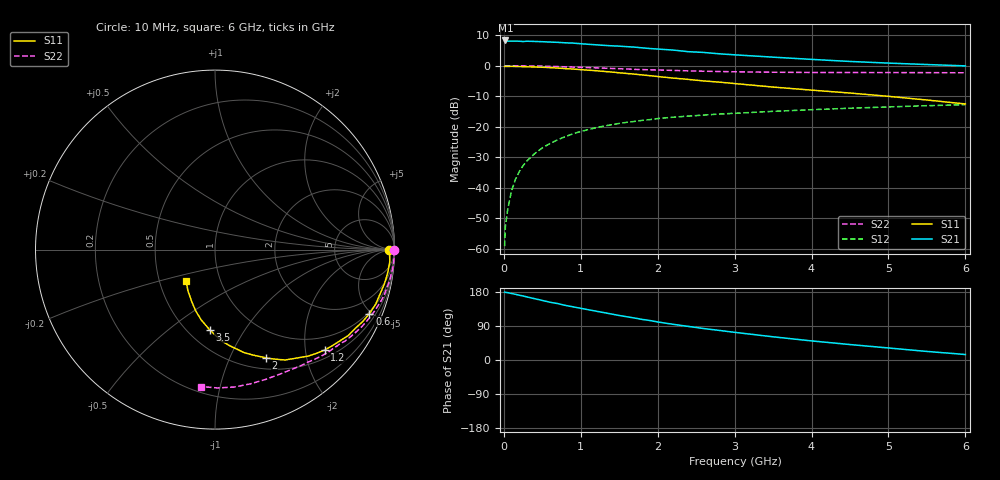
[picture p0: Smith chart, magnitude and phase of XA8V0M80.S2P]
! SIEMENS Discrete & RF Semiconductors
! BFY180
! Si NPN RF Bipolar Junction Transistor in MICRO-X
! VCE = 8 V  IC = 0.8 mA
! Common Emitter S-Parameters:  May  1997
# GHz  S  MA  R  50
!  f  S11  S21  S12  S22
! GHz  MAG  ANG  MAG  ANG  MAG  ANG  MAG  ANG
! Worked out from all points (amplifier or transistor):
!   36 points, 10 MHz to 6 GHz, reference 50 ohm
!   highest |S21| = 8.3 dB at 20 MHz (marker M1)
!   |S21| within 3 dB of that: start of sweep to 2.109 GHz
!   unconditionally stable (mu >= 1): 4.863 GHz to end of sweep
!   at 250 MHz: K = 0.06, MSG = 20.4 dB, |S12| = -32.8 dB
!   at 1.4 GHz: K = 0.44, MSG = 12.9 dB, |S12| = -19.3 dB
!   at 6 GHz: K = 1.03, MAG = 5.3 dB, |S12| = -12.8 dB
!   S11 on the Smith chart (normalised r, x): 10 MHz: 68, -8; 600 MHz: 0.91, -4.86; 1.2 GHz: 0.68, -2.42; 2 GHz: 0.63, -1.37; 3.5 GHz: 0.63, -0.71; 6 GHz: 0.68, -0.25
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0.01  0.9716 -0.2  2.527 179.2  0.0011 93.7  0.9981 -0.2
0.02  0.9765 -0.8  2.599 178.5  0.0023 86.0  0.9999 -0.5
0.05  0.9735 -1.9  2.538 177.7  0.0044 87.1  0.9976 -1.2
0.1  0.9763 -3.8  2.53 175.5  0.0089 87.9  0.998 -2.5
0.15  0.9729 -5.9  2.538 173.4  0.0136 87.0  0.9978 -3.7
0.2  0.9713 -7.4  2.524 170.9  0.0183 84.1  0.997 -4.9
0.3  0.9633 -11.3  2.526 166.4  0.0275 81.6  0.9926 -7.3
0.4  0.9519 -15.3  2.505 161.8  0.0361 79.8  0.9892 -9.8
0.6  0.9312 -22.5  2.448 152.4  0.053 74.0  0.9768 -14.5
0.9  0.8835 -32.8  2.353 140.3  0.0766 65.5  0.9518 -21.3
1.1  0.8454 -39.2  2.248 132.6  0.09 61.0  0.9332 -25.5
1.2  0.8291 -42.4  2.205 128.8  0.0966 58.7  0.9243 -27.6
1.6  0.7467 -54.5  2.056 114.1  0.1182 51.0  0.8852 -35.2
2  0.6655 -64.9  1.879 100.4  0.136 44.3  0.8528 -41.8
2.2  0.628 -69.7  1.808 94.2  0.1433 41.2  0.8385 -45.0
2.6  0.5634 -78.2  1.653 83.0  0.1553 36.3  0.8129 -50.6
3  0.5105 -85.9  1.511 73.0  0.1661 31.8  0.7964 -56.0
3.5  0.4471 -93.9  1.383 61.2  0.1788 27.1  0.7828 -62.3
4  0.3984 -101.2  1.272 50.4  0.1902 22.6  0.7762 -68.7
4.5  0.3568 -107.7  1.176 40.8  0.2012 18.4  0.7735 -75.3
5.5  0.2742 -123.4  1.047 22.6  0.2213 10.1  0.771 -88.9
6  0.2364 -133.1  0.995 14.5  0.2298 5.7  0.7668 -95.8
